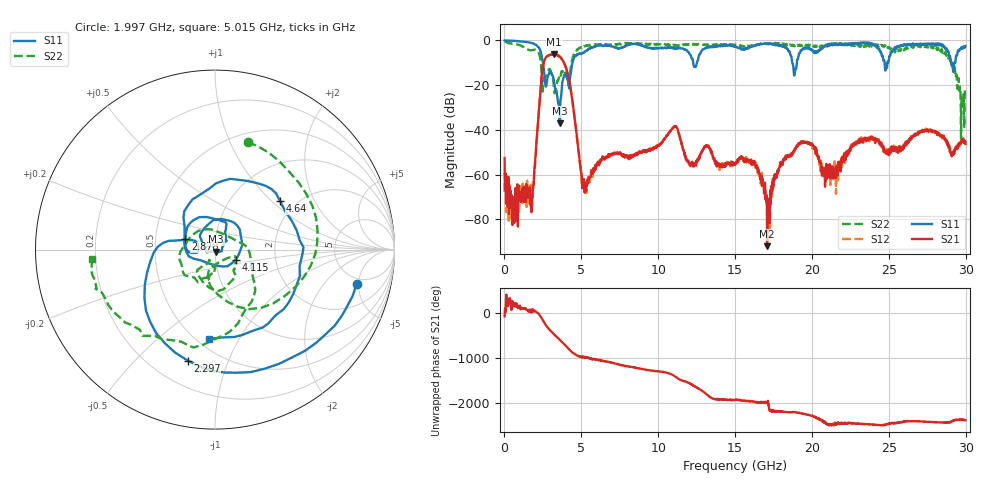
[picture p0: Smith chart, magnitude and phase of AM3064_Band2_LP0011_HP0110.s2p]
# Hz S DB R 50.0
!freq dBS11 angS11 dBS21 angS21 dBS12 angS12 dBS22 angS22
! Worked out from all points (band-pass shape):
!   1600 points, 10 MHz to 29.98 GHz, reference 50 ohm
!   highest |S21| = -6.12 dB at 3.234 GHz (marker M1); lowest = -91.9 dB at 17.09 GHz (marker M2)
!   |S21| within 3 dB of the highest: 2.59 GHz to 3.808 GHz (1.218 GHz wide, 38.1 % of centre)
!   lowest |S11| = -37.1 dB at 3.59 GHz (marker M3), VSWR 1.03, Z = 50.6 - j1.25 ohm
!   |S11| at or under -10 dB: 2.505 GHz to 4.432 GHz (1.927 GHz wide, 55.6 % of centre); 18.72 GHz to 19.02 GHz (295.6 MHz wide, 1.57 % of centre); 29.04 GHz to 29.29 GHz (242.4 MHz wide, 0.831 % of centre)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
!   |S22| runs from -45.8 to -0.2 dB; largest |S21 - S12| = 0.018
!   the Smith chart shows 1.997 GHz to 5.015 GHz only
!   S11 on the Smith chart (normalised r, x): 1.997 GHz: 4.19, -4.73; 2.297 GHz: 0.35, -0.72; 2.878 GHz: 0.71, +0.08; 4.115 GHz: 1.25, -0.15; 4.64 GHz: 1.65, +1.13; 5.015 GHz: 0.57, -0.76
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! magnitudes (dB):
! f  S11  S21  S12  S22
! 10 MHz  0.0  -52.6  -67.6  -0.2
! 647.3 MHz  -0.3  -81.3  -71.6  -1.6
! 1.753 GHz  -1.1  -76.7  -73.1  -4.3
! 1.997 GHz  -1.8  -53.9  -54.0  -4.1
! 2.297 GHz  -3.9  -25.9  -26.0  -7.1
! 2.878 GHz  -15.2  -6.7  -6.6  -13.1
! 3.234 GHz  -19.1  -6.1  -6.3  -22.6
! 3.59 GHz  -37.1  -7.3  -7.3  -15.2
! 4.115 GHz  -17.8  -14.9  -14.7  -18.4
! 4.64 GHz  -6.9  -38.9  -38.9  -5.2
! 5.015 GHz  -6.1  -59.8  -62.8  -3.3
! 10 GHz  -3.5  -47.1  -47.2  -1.8
! 11.11 GHz  -3.9  -38.6  -38.4  -2.3
! 15 GHz  -2.6  -55.1  -55.3  -1.8
! 16.28 GHz  -2.2  -54.6  -54.7  -2.2
! 17.09 GHz  -1.6  -91.9  -74.5  -1.5
! 18.25 GHz  -3.3  -52.7  -53.5  -1.8
! 19.99 GHz  -4.1  -46.1  -47.0  -2.1
! 20.82 GHz  -2.6  -60.9  -57.9  -2.3
! 25 GHz  -9.1  -51.0  -48.6  -2.9
! 28.56 GHz  -2.6  -43.5  -43.5  -4.7
! 29.98 GHz  -2.5  -46.3  -45.3  -21.5
